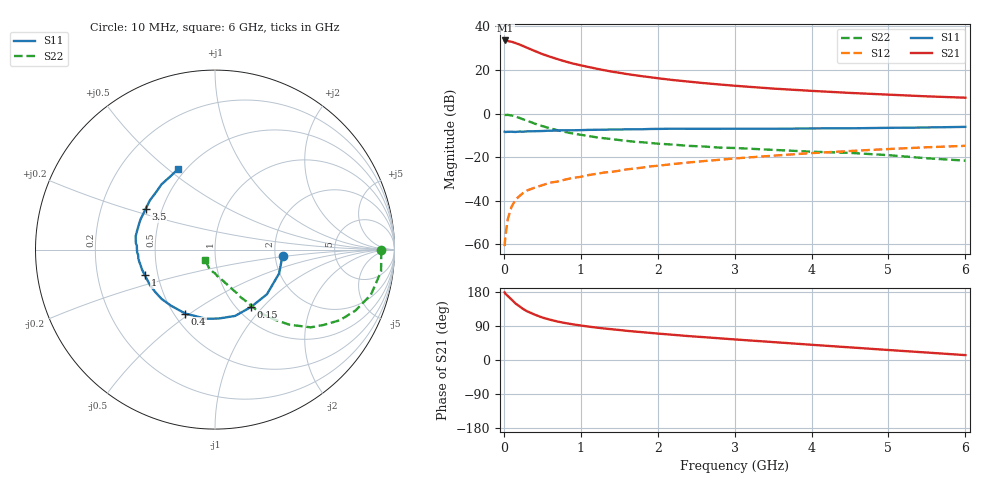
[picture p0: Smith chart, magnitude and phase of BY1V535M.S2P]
! SIEMENS Small Signal Semiconductors
! BFY420
! Si NPN RF SIEGET Grounded Emitter Transistor in MICRO-X
! VCE = 1.5 V  IC = 35 mA
! Common Emitter S-Parameters:  October  1996
# GHz  S  MA  R  50
!  f  S11  S21  S12  S22
! GHz  MAG  ANG  MAG  ANG  MAG  ANG  MAG  ANG
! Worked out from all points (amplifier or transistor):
!   36 points, 10 MHz to 6 GHz, reference 50 ohm
!   highest |S21| = 33.6 dB at 20 MHz (marker M1)
!   |S21| within 3 dB of that: start of sweep to 278.6 MHz
!   unconditionally stable (mu >= 1): start of sweep to 16.15 MHz; 1.374 GHz to end of sweep
!   at 250 MHz: K = 0.41, MSG = 33.7 dB, |S12| = -36.5 dB
!   at 1.4 GHz: K = 1.01, MAG = 22.4 dB, |S12| = -26.8 dB
!   at 6 GHz: K = 1.08, MAG = 9.3 dB, |S12| = -14.8 dB
!   S11 on the Smith chart (normalised r, x): 10 MHz: 2.22, -0.18; 150 MHz: 1.16, -0.86; 400 MHz: 0.57, -0.48; 1 GHz: 0.42, -0.15; 3.5 GHz: 0.40, +0.23; 6 GHz: 0.46, +0.55
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0.01  0.3827 -5.2  47.65 178.5  0.0009 120.9  0.9228 -0.3
0.02  0.376 -9.2  47.7 175.1  0.0015 82.8  0.9268 -2.0
0.05  0.3811 -20.5  46.23 169.1  0.0037 81.4  0.9332 -7.5
0.1  0.3816 -40.7  44.59 159.6  0.0072 73.7  0.9045 -16.1
0.15  0.3774 -57.9  41.62 149.5  0.0104 71.8  0.8536 -23.4
0.2  0.3861 -73.1  38.74 142.1  0.0126 70.1  0.7993 -29.5
0.25  0.3845 -86.8  35.49 134.7  0.015 65.1  0.7371 -34.7
0.3  0.3884 -97.5  32.53 128.8  0.017 63.2  0.6867 -39.1
0.4  0.3928 -114.9  27.42 119.8  0.0199 61.6  0.5885 -45.3
0.5  0.3969 -127.9  23.22 112.1  0.0226 60.3  0.5145 -49.5
0.6  0.4051 -137.2  20.17 106.4  0.0258 60.6  0.4578 -52.8
0.7  0.408 -144.3  17.73 101.4  0.0275 60.3  0.4137 -55.2
0.8  0.4126 -151.0  15.69 97.4  0.0305 59.4  0.3763 -57.1
1  0.4158 -159.8  12.79 91.0  0.0353 61.4  0.325 -59.7
1.1  0.4215 -164.7  11.73 88.2  0.0386 61.6  0.3045 -61.5
1.4  0.4301 -173.6  9.195 81.2  0.0458 61.6  0.2593 -64.5
1.6  0.4341 -178.0  8.067 77.0  0.0523 61.0  0.2351 -66.9
2.2  0.4483 170.5  5.883 66.5  0.0692 58.6  0.1937 -73.0
3.5  0.4478 149.8  3.744 47.3  0.1077 49.6  0.1466 -85.5
4.5  0.4578 136.3  2.977 33.3  0.138 40.7  0.125 -95.4
5.5  0.4785 120.9  2.482 19.7  0.1681 30.8  0.0939 -116.6
6  0.4944 114.3  2.312 12.9  0.1815 25.6  0.0829 -133.9
